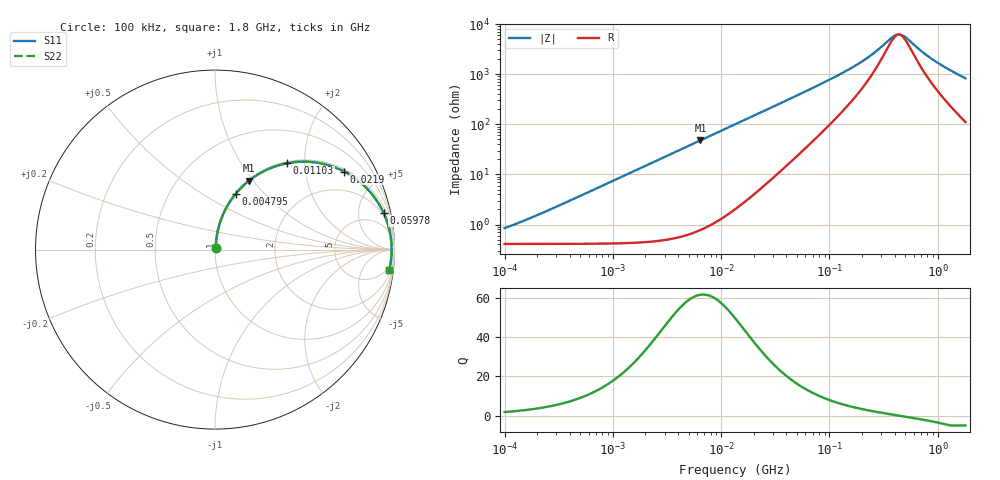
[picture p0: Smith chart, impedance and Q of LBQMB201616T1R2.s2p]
! LBQMB201616T1R2  S-PARAMETER MODEL  ( General Type )
! Model Generated by TAIYO YUDEN Corporation (http://www.ty-top.com)
! Version 1.0
! TAIYO YUDEN Control No. 191025NI43SB-FBB
! Copyright(c) 2019 TAIYO YUDEN CO.,LTD. All Rights Reserved.
! Product Description (link to TY-COMPAS)
! https://ds.yuden.co.jp/TYCOMPAS/or/detail?pn=LBQMB201616T1R2J&u=M
! Products Name : Inductors
! Characteristics :
!  Inductance : 1.2 uH , SRF(min) : 180 MHz , DC Resistance(max) : 0.533 Ohm , Rated Current : 370 mA
!  Case Size : 2.0 x 1.6 / 0.079 x 0.063 [mm/inch] , Thickness : 1.6 / 0.063 [mm/inch]
!  (Conditions: Temperature = 25 degC , DC Bias Current/Voltage = 0A / 0V)
! External Node Assignments :
!  1  o---GGG---o  2
! GND o---------o GND
! Frequency Range : 0.1MHz  -  1800MHz  [ 402 STEP ]
# MHz S RI R 50
! Freq[MHz].  S11 Real  S11 Imag  S21 Real  S21 Imag  S12 Real  S12 Imag  S22 Real  S22 Imag
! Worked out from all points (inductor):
!   401 points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, 100 kHz to 1.8 GHz, reference 50 ohm
!   read as one part in series: L = 1.18 uH near 167.3 kHz
!   highest Q = 61.4 at 6.434 MHz (marker M1), where L = 1.18 uH
!   self-resonance near 437.1 MHz
!   S11 on the Smith chart (normalised r, x): 100 kHz: 1.01, +0.01; 4.795 MHz: 1.01, +0.71; 11.03 MHz: 1.03, +1.64; 21.9 MHz: 1.09, +3.25; 59.78 MHz: 1.66, +8.99; 1.8 GHz: 3, -16
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0.1  0.00414 0.00735  0.9959 -0.00735  0.9959 -0.00735  0.00414 0.00735
0.180018  0.00426 0.0132  0.9957 -0.0132  0.9957 -0.0132  0.00426 0.0132
0.516129  0.00555 0.0379  0.9944 -0.0379  0.9944 -0.0379  0.00555 0.0379
1.277529  0.013 0.0931  0.987 -0.0931  0.987 -0.0931  0.013 0.0931
2.66389  0.0417 0.1884  0.9583 -0.1884  0.9583 -0.1884  0.0417 0.1884
4.795486  0.1165 0.3123  0.8835 -0.3123  0.8835 -0.3123  0.1165 0.3123
6.434145  0.1894 0.3838  0.8106 -0.3838  0.8106 -0.3838  0.1894 0.3838
11.02886  0.4027 0.4814  0.5973 -0.4814  0.5973 -0.4814  0.4027 0.4814
13.41641  0.4978 0.49  0.5022 -0.49  0.5022 -0.49  0.4978 0.49
21.89777  0.7202 0.4347  0.2798 -0.4347  0.2798 -0.4347  0.7202 0.4347
34.87589  0.8606 0.3252  0.1394 -0.3252  0.1394 -0.3252  0.8606 0.3252
59.78129  0.9394 0.2046  0.0606 -0.2046  0.0606 -0.2046  0.9394 0.2046
69.24595  0.9508 0.1776  0.0492 -0.1776  0.0492 -0.1776  0.9508 0.1776
124.6553  0.9748 0.0953  0.0252 -0.0953  0.0252 -0.0953  0.9748 0.0953
189.0427  0.9809 0.056  0.0191 -0.056  0.0191 -0.056  0.9809 0.056
259.9299  0.9831 0.0324  0.0169 -0.0324  0.0169 -0.0324  0.9831 0.0324
357.3983  0.984 0.0121  0.016 -0.0121  0.016 -0.0121  0.984 0.0121
413.9822  0.9841 0.00325  0.0159 -0.00325  0.0159 -0.00325  0.9841 0.00325
479.5244  0.9841 -0.00555  0.0159 0.00555  0.0159 0.00555  0.9841 -0.00555
906.5744  0.9818 -0.0475  0.0182 0.0475  0.0182 0.0475  0.9818 -0.0475
1277.433  0.9781 -0.0766  0.0219 0.0766  0.0219 0.0766  0.9781 -0.0766
1800  0.9706 -0.1142  0.0294 0.1142  0.0294 0.1142  0.9706 -0.1142
